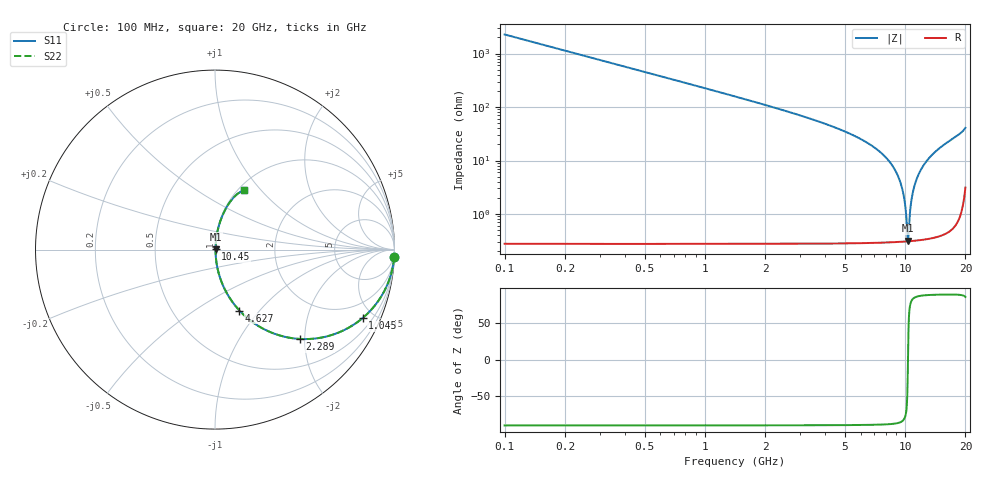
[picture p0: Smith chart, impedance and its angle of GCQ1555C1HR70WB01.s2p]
!Murata Part Number: GCQ1555C1HR70WB01
!These Parameters are Measured in Series Mode Connection
!Data Generated on Jan 08, 2026
!  o--ll--o
!Port1  Port2
!  o------o
!Operation Temp=25[degC], DC Bias Voltage=0[V]
!Freq. Start=100[MHz] Stop=20[GHz] 401[Steps]
# Hz S RI R 50
!Freq.(Hz) S11(Real) S11(Imag) S21(Real) S21(Imag) S12(Real) S12(Imag) S22(Real) S22(Imag)
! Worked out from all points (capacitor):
!   401 points, 100 MHz to 20 GHz, reference 50 ohm
!   read as one part in series: C = 700 fF near 199.5 MHz
!   lowest |Z| = 315 mohm at 10.35 GHz (marker M1)
!   series resonance near 10.33 GHz, so ESL is about 340 pH
!   S11 on the Smith chart (normalised r, x): 100 MHz: 1, -45; 1.045 GHz: 1.01, -4.31; 2.289 GHz: 1.01, -1.89; 4.627 GHz: 1.01, -0.79; 10.45 GHz: 1.01, +0.01; 20 GHz: 1.06, +0.82
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1e8  0.9981 -0.0439  0.00194 0.0439  0.00194 0.0439  0.9981 -0.0439
2.99e8  0.9829 -0.1294  0.0171 0.1294  0.0171 0.1294  0.9829 -0.1294
4.4825e8  0.9624 -0.1901  0.0376 0.1901  0.0376 0.1901  0.9624 -0.1901
1.04525e9  0.8223 -0.3816  0.1777 0.3816  0.1777 0.3816  0.8223 -0.3816
2.289e9  0.4719 -0.4977  0.5281 0.4977  0.5281 0.4977  0.4719 -0.4977
3.43325e9  0.2592 -0.4358  0.7408 0.4358  0.7408 0.4358  0.2592 -0.4358
4.62725e9  0.1361 -0.3393  0.8639 0.3393  0.8639 0.3393  0.1361 -0.3393
6.7665e9  0.0385 -0.1851  0.9615 0.1851  0.9615 0.1851  0.0385 -0.1851
8.10975e9  0.0145 -0.1068  0.9855 0.1068  0.9855 0.1068  0.0145 -0.1068
9.055e9  0.00641 -0.0584  0.9936 0.0584  0.9936 0.0584  0.00641 -0.0584
9.652e9  0.00394 -0.0302  0.9961 0.0302  0.9961 0.0302  0.00394 -0.0302
1.005e10  0.0032 -0.0124  0.9968 0.0124  0.9968 0.0124  0.0032 -0.0124
1.0249e10  0.00308 -0.00366  0.9969 0.00366  0.9969 0.00366  0.00308 -0.00366
1.03485e10  0.00308 0.000632  0.9969 -0.000632  0.9969 -0.000632  0.00308 0.000632
1.0448e10  0.00311 0.00488  0.9969 -0.00488  0.9969 -0.00488  0.00311 0.00488
1.059725e10  0.00322 0.0112  0.9968 -0.0112  0.9968 -0.0112  0.00322 0.0112
1.07465e10  0.00342 0.0174  0.9966 -0.0174  0.9966 -0.0174  0.00342 0.0174
1.1244e10  0.00458 0.0376  0.9954 -0.0376  0.9954 -0.0376  0.00458 0.0376
1.208975e10  0.00822 0.0702  0.9918 -0.0702  0.9918 -0.0702  0.00822 0.0702
1.338325e10  0.0172 0.1162  0.9828 -0.1162  0.9828 -0.1162  0.0172 0.1162
1.67165e10  0.0564 0.2209  0.9436 -0.2209  0.9436 -0.2209  0.0564 0.2209
2e10  0.1613 0.3315  0.8387 -0.3315  0.8387 -0.3315  0.1613 0.3315
